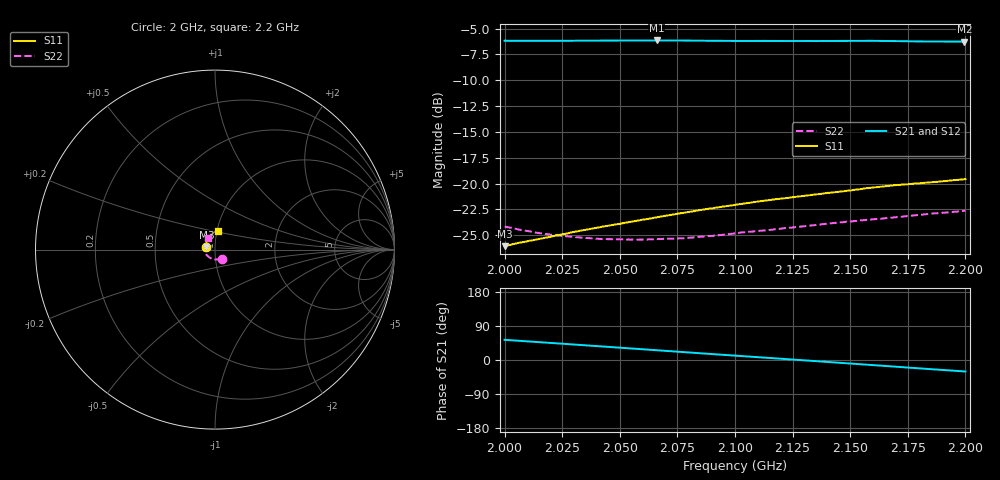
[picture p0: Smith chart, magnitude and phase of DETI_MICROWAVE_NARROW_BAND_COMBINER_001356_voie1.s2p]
! 12/28/2020 4:20:30 PM
! \\DETI-AD\SERVEUR COMMUN\0\01 - PRODUIT\0 01 356 - COMBINEUR 4 VOIES BANDE S 800 WATTS\81 -PROCES VERBAL DE CONTROLE\MESURES\07 - S2P\VOIE1.S2P
! CHANNEL.1
! TR.MEASUREMENT
! CORRECTED.DATA
# GHZ S RI R 50.0
! FREQ.GHZ  S11RE  S11IM  S21RE  S21IM  S12RE  S12IM  S22RE  S22IM
!; PortSelection: Port_12
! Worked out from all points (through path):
!   1000 points, 2 GHz to 2.2 GHz, reference 50 ohm
!   highest |S21| = -6.15 dB at 2.066 GHz (marker M1); lowest = -6.3 dB at 2.2 GHz (marker M2)
!   lowest |S11| = -26.1 dB at 2 GHz (marker M3), VSWR 1.10, Z = 45.4 + j1.34 ohm
!   |S11| at or under -10 dB: start of sweep to end of sweep
!   |S22| runs from -25.4 to -22.6 dB; largest |S21 - S12| = 0.002
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2  -0.0477 0.0144  0.2937 0.3935  0.2938 0.3939  0.0368 -0.0497
2.0002  -0.0476 0.0147  0.2946 0.3929  0.2942 0.3936  0.0366 -0.0498
2.006006  -0.0485 0.0178  0.3107 0.3802  0.3105 0.3807  0.0302 -0.0518
2.016617  -0.0488 0.0239  0.3383 0.3554  0.3387 0.3556  0.0183 -0.0542
2.024424  -0.0491 0.0282  0.3579 0.3358  0.3582 0.3359  0.00974 -0.055
2.033433  -0.0492 0.0333  0.3793 0.3121  0.3798 0.3117  6.43e-05 -0.0547
2.042042  -0.0487 0.038  0.3984 0.2881  0.3988 0.2876  -0.00887 -0.0532
2.045846  -0.0482 0.0401  0.4065 0.2771  0.4066 0.2765  -0.0128 -0.0523
2.057257  -0.047 0.0464  0.4286 0.2421  0.4285 0.2414  -0.0237 -0.048
2.066066  -0.0456 0.0514  0.4437 0.2139  0.443 0.2133  -0.0317 -0.0436
2.066667  -0.0456 0.0517  0.4446 0.2119  0.444 0.2113  -0.0321 -0.0433
2.077678  -0.0433 0.0578  0.4598 0.1749  0.4593 0.1747  -0.0405 -0.0363
2.08989  -0.04 0.0644  0.4725 0.1327  0.4722 0.1325  -0.0486 -0.0275
2.1001  -0.0369 0.0697  0.4803 0.097  0.4804 0.097  -0.0542 -0.0193
2.114515  -0.0316 0.0769  0.4876 0.0473  0.4877 0.0468  -0.0593 -0.00678
2.133534  -0.023 0.0851  0.4892 -0.0197  0.4885 -0.0211  -0.0619 0.0105
2.144945  -0.0172 0.0896  0.4863 -0.0614  0.4851 -0.0624  -0.0612 0.0209
2.152553  -0.0128 0.0926  0.4825 -0.0886  0.481 -0.0891  -0.0598 0.0278
2.166767  -0.00448 0.0974  0.4698 -0.1381  0.4679 -0.1377  -0.0551 0.0403
2.187788  0.0104 0.1015  0.4397 -0.2086  0.4394 -0.208  -0.0446 0.0565
2.1996  0.0192 0.1032  0.4201 -0.2442  0.4201 -0.2441  -0.0368 0.0641
2.2  0.0195 0.1032  0.4195 -0.2456  0.4195 -0.2454  -0.0364 0.0644
